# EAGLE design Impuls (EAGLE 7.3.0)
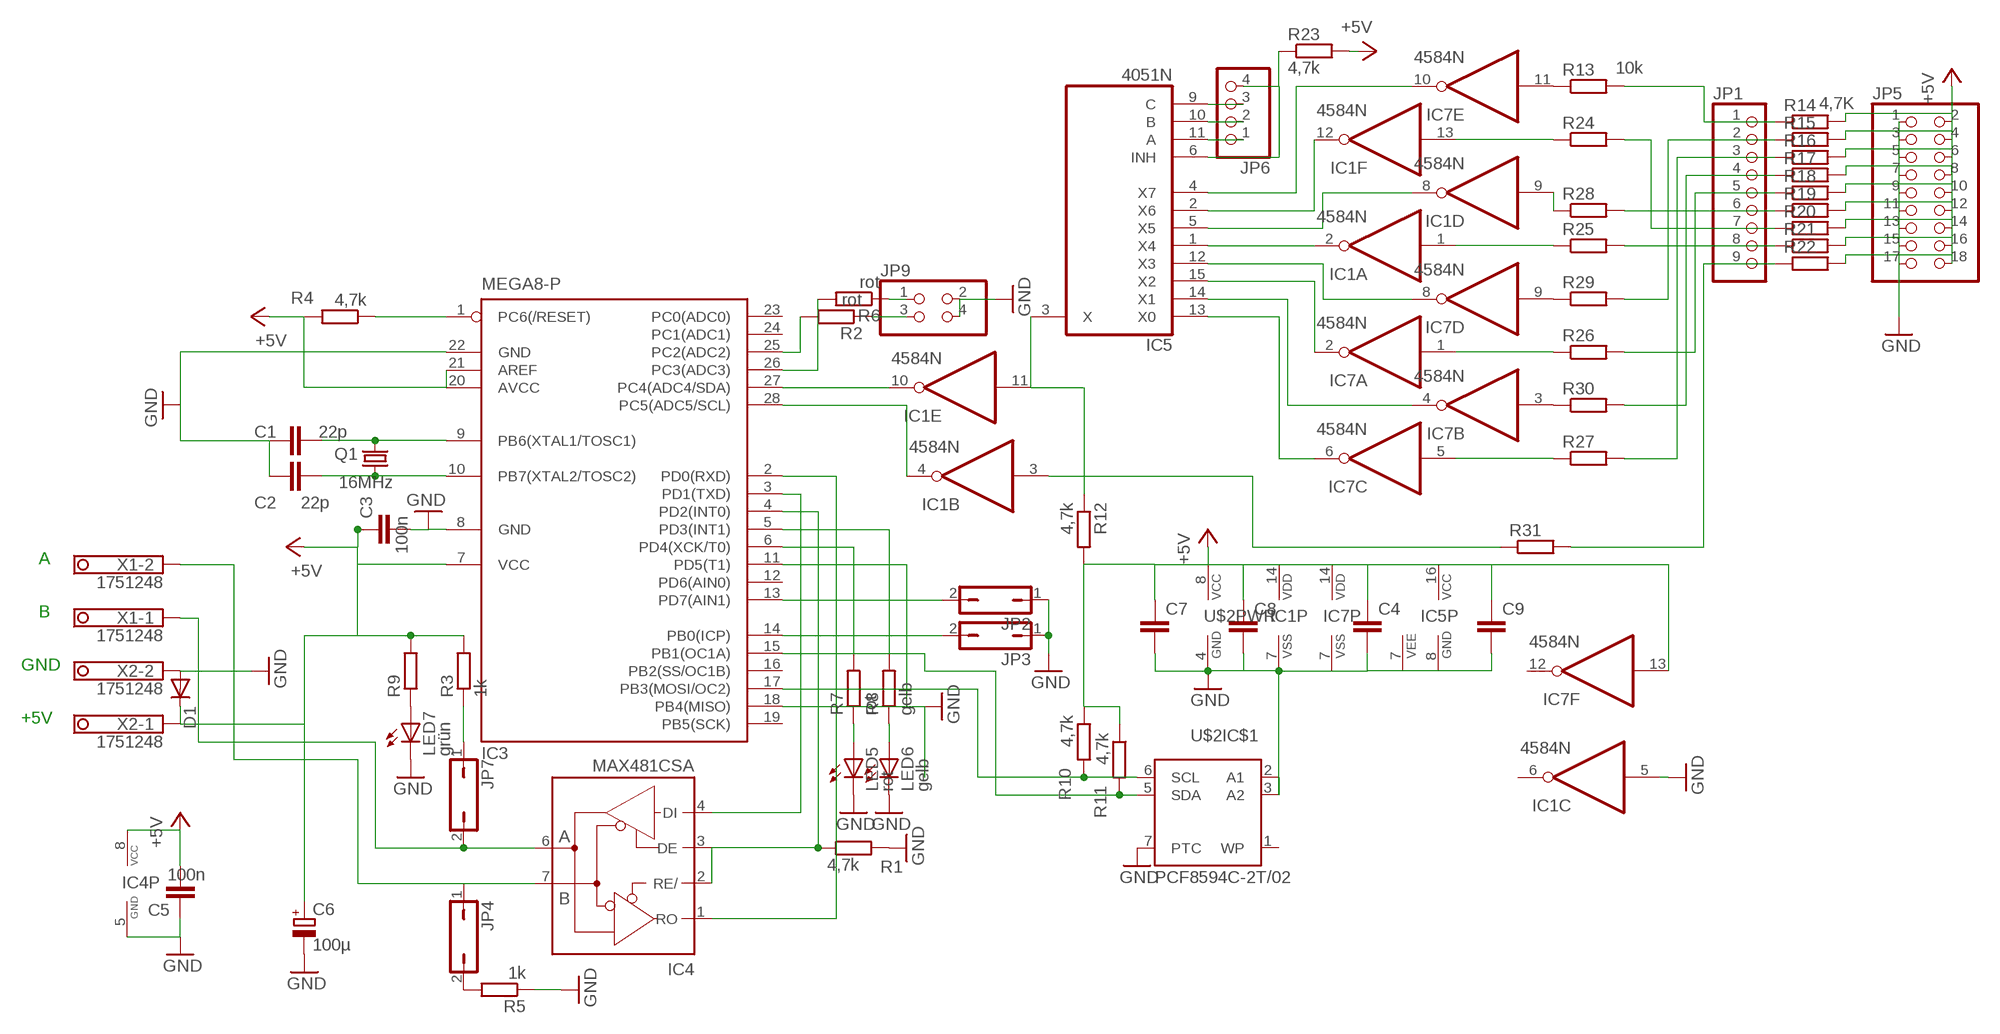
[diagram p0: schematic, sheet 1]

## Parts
C1  22p  C-EUC0603  [C0603]
C2  22p  C-EUC0603  [C0603]
C3  100n  C-EUC0603  [C0603]
C4  C-EUC0603  [C0603]
C5  100n  C-EUC0603  [C0603]
C6  100µ  CPOL-EUSMCD  [SMC_D]
C7  C-EUC0603  [C0603]
C8  C-EUC0603  [C0603]
C9  C-EUC0603  [C0603]
D1  DIODE-DO214AA  [DO214AA]
IC1  4584N  [DIL14]
IC3  MEGA8-P  [DIL28-3]
IC4  MAX481CSA  [SO08]
IC5  4051N  [DIL16]
IC7  4584N  [DIL14]
JP1  PINHD-1X9  [1X09]
JP2  JP1Q  [JP1]
JP3  JP1Q  [JP1]
JP4  JP1Q  [JP1]
JP5  PINHD-2X9  [2X09]
JP6  PINHD-1X4  [1X04]
JP7  JP1Q  [JP1]
JP9  PINHD-2X2  [2X02]
LED5  rot  LED3MM  [LED3MM]
LED6  gelb  LED3MM  [LED3MM]
LED7  grün  LED3MM  [LED3MM]
Q1  16MHz  CRYSTALCTS406  [CTS406]
R1  4,7k  R-EU_R0603  [R0603]
R2  rot  R-EU_R0603  [R0603]
R3  1k  R-EU_R0603  [R0603]
R4  4,7k  R-EU_R0603  [R0603]
R5  1k  R-EU_R0603  [R0603]
R6  rot  R-EU_R0603  [R0603]
R7  rot  R-EU_R0603  [R0603]
R8  gelb  R-EU_R0603  [R0603]
R9  R-EU_R0603  [R0603]
R10  4,7k  R-EU_R0603  [R0603]
R11  4,7k  R-EU_R0603  [R0603]
R12  4,7k  R-EU_R0603  [R0603]
R13  10k  R-EU_R0603  [R0603]
R14  4,7K  R-EU_R0603  [R0603]
R15  R-EU_R0603  [R0603]
R16  R-EU_R0603  [R0603]
R17  R-EU_R0603  [R0603]
R18  R-EU_R0603  [R0603]
R19  R-EU_R0603  [R0603]
R20  R-EU_R0603  [R0603]
R21  R-EU_R0603  [R0603]
R22  R-EU_R0603  [R0603]
R23  4,7k  R-EU_R0603  [R0603]
R24  R-EU_R0603  [R0603]
R25  R-EU_R0603  [R0603]
R26  R-EU_R0603  [R0603]
R27  R-EU_R0603  [R0603]
R28  R-EU_R0603  [R0603]
R29  R-EU_R0603  [R0603]
R30  R-EU_R0603  [R0603]
R31  R-EU_R0603  [R0603]
U$2  PCF8594C-2T/02  [SO08]
X1  1751248  [1751248]
X2  1751248  [1751248]

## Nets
+5V: C3.1 C4.1 C5.2 C6.+ C7.1 C8.1 C9.1 D1.C IC1.14(P:VDD) IC3.7(VCC) IC3.20(AVCC) IC3.21(AREF) IC4.8(VCC) IC5.16(VCC) IC7.13(F:I) IC7.14(P:VDD) JP5.2 JP5.4 JP5.6 JP5.8 JP5.10 JP5.12 JP5.14 JP5.16 JP5.18 R3.2 R4.2 R9.2 R10.1 R11.1 R12.2 R14.2 R15.2 R16.2 R17.2 R18.2 R19.2 R20.2 R21.2 R22.2 R23.2 U$2.8(PWR:VCC) X2.1
GND: C1.1 C2.1 C3.2 C4.2 C5.1 C6.- C7.2 C8.2 C9.2 D1.A IC1.5(C:I) IC1.7(P:VSS) IC3.8(GND) IC3.11(PD5(T1)) IC3.18(PB4(MISO)) IC3.22(GND) IC4.5(GND) IC5.7(VEE) IC5.8(GND) IC7.7(P:VSS) JP2.1 JP3.1 JP5.1 JP5.3 JP5.5 JP5.7 JP5.9 JP5.11 JP5.13 JP5.15 JP5.17 JP9.2 JP9.4 LED5.K(C) LED6.K(C) LED7.K(C) R1.2 R5.1 U$2.2(IC$1:A1) U$2.3(IC$1:A2) U$2.4(PWR:GND) U$2.7(IC$1:PTC) X2.2
N$1: IC1.4(B:O) IC3.28(PC5(ADC5/SCL))
N$2: IC3.2(PD0(RXD)) IC4.1(RO)
N$3: IC4.6(A) JP7.2 X1.1
N$4: IC4.7(B) JP4.1 X1.2
N$5: IC3.17(PB3(MOSI/OC2)) R10.2 U$2.6(IC$1:SCL)
N$6: IC3.13(PD7(AIN1)) JP2.2
N$7: IC3.15(PB1(OC1A)) R11.2 U$2.5(IC$1:SDA)
N$8: LED7.A R9.1
N$9: IC3.26(PC3(ADC3)) R6.2
N$10: IC3.1(PC6(/RESET)) R4.1
N$11: C2.2 IC3.10(PB7(XTAL2/TOSC2)) Q1.1
N$12: C1.2 IC3.9(PB6(XTAL1/TOSC1)) Q1.3
N$13: IC3.3(PD1(TXD)) IC4.4(DI)
N$14: IC3.14(PB0(ICP)) JP3.2
N$15: IC3.4(PD2(INT0)) IC4.2(RE/) IC4.3(DE) R1.1
N$16: IC3.25(PC2(ADC2)) R2.2
N$17: JP9.3 R2.1
N$18: JP9.1 R6.1
N$19: IC1.10(E:O) IC3.27(PC4(ADC4/SDA))
N$21: IC5.15(X2) IC7.2(A:O)
N$22: IC5.11(A) JP6.1
N$23: IC5.10(B) JP6.2
N$24: IC5.9(C) JP6.3
N$25: IC1.3(B:I) R31.1
N$26: IC1.2(A:O) IC5.1(X4)
N$27: IC1.12(F:O) IC5.2(X6)
N$28: IC1.8(D:O) IC5.5(X5)
N$29: IC5.4(X7) IC7.10(E:O)
N$30: IC5.13(X0) IC7.6(C:O)
N$31: IC5.14(X1) IC7.4(B:O)
N$32: JP1.8 R21.1 R25.2
N$33: IC5.12(X3) IC7.8(D:O)
N$34: IC1.11(E:I) IC5.3(X) R12.1
N$35: JP1.7 R20.1 R24.2
N$36: IC3.6(PD4(XCK/T0)) R7.2
N$37: IC3.5(PD3(INT1)) R8.2
N$38: LED5.A R7.1
N$39: LED6.A R8.1
N$40: JP1.6 R19.1 R28.2
N$41: JP1.5 R18.1 R26.2
N$42: JP1.4 R17.1 R30.2
N$43: IC1.9(D:I) R28.1
N$44: JP1.2 R15.1 R29.2
N$45: IC5.6(INH) JP6.4 R23.1
N$46: IC7.11(E:I) R13.1
N$47: IC1.13(F:I) R24.1
N$48: IC1.1(A:I) R25.1
N$49: IC7.1(A:I) R26.1
N$50: IC7.5(C:I) R27.1
N$51: JP1.3 R16.1 R27.2
N$52: IC7.3(B:I) R30.1
N$53: IC7.9(D:I) R29.1
N$54: JP1.9 R22.1 R31.2
N$55: JP1.1 R13.2 R14.1
N$56: JP4.2 R5.2
N$57: JP7.1 R3.1
Unconnected: IC1.6(C:O) IC3.12(PD6(AIN0)) IC3.16(PB2(SS/OC1B)) IC3.19(PB5(SCK)) IC3.23(PC0(ADC0)) IC3.24(PC1(ADC1)) IC7.12(F:O) U$2.1(IC$1:WP)

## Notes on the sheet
- A
- B
- GND
- +5V

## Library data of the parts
C1-C5 C7-C9 = rcl:C-EU: CAPACITOR, European symbol
C6 = rcl:CPOL-EU: POLARIZED CAPACITOR, European symbol
D1 = diode:DIODE-: DIODE
IC1 IC7 = 45xx:4584: Hex SCHMITT TRIGGER (74C14)
IC3 = atmel:MEGA8-P: MICROCONTROLLER 8 Kbytes FLASH, 1 kbytes SRAM, 512 bytes EEPROM, USART, 4-channel 10 bit ADC, 2-channel 8 bit ADC Pin compatible with Atmega48, ATMega88, ATMega168 Source: avr.lbr
IC4 = maxim:MAX481CSA: RS485 TRANSEIVER
IC5 = 40xx:4051: 8-channel ANALOG MULTIPLEXER
JP1 = pinhead:PINHD-1X9: PIN HEADER
JP2-JP4 JP7 = jumper:JP1Q: JUMPER
JP5 = pinhead:PINHD-2X9: PIN HEADER
JP6 = pinhead:PINHD-1X4: PIN HEADER
JP9 = pinhead:PINHD-2X2: PIN HEADER
LED5-LED7 = led:LED: LED
Q1 = crystal:CRYSTAL: CRYSTAL
R1-R31 = rcl:R-EU_: RESISTOR, European symbol
U$2 = i2c:PCF8594C-2: 512 x 8-Bit CMOS EEPROM with I²C Bus Interface
X1 X2 = con-phoenix-350:1751248: MKDS 1/ 2-3,5 Printklemme

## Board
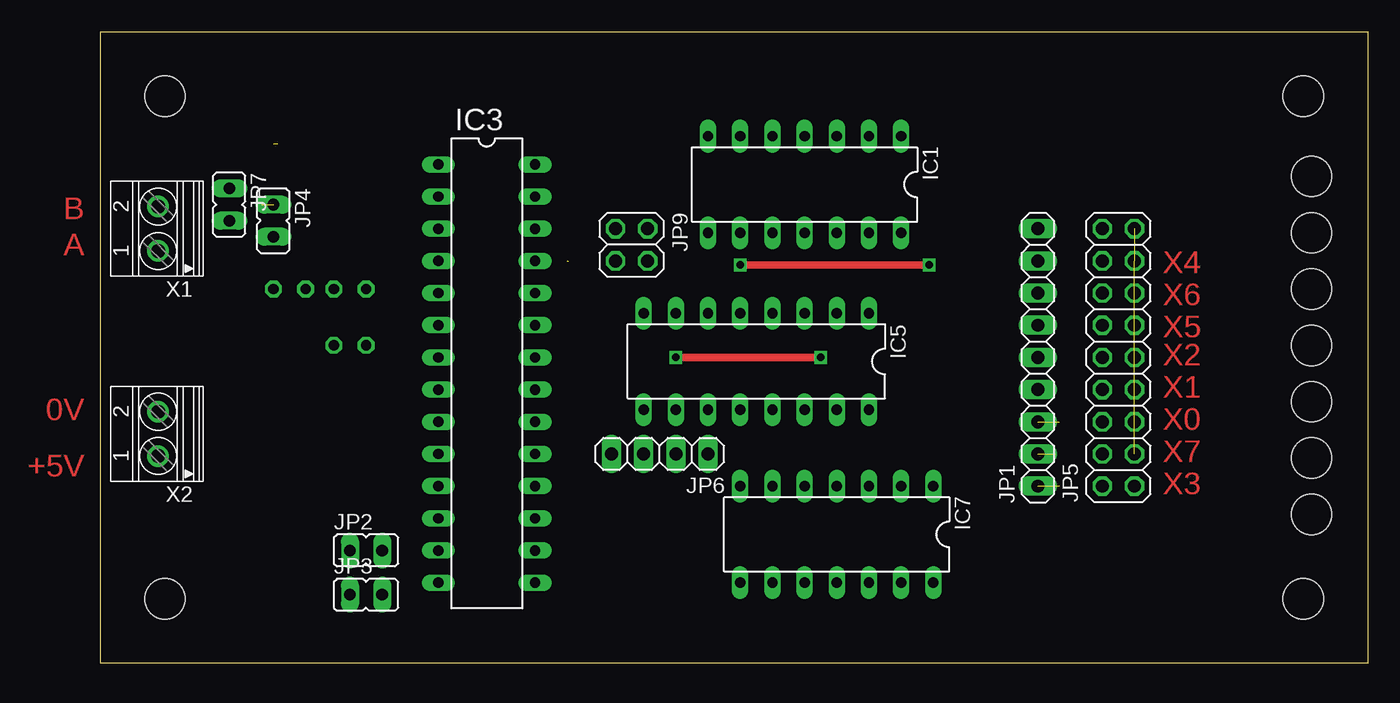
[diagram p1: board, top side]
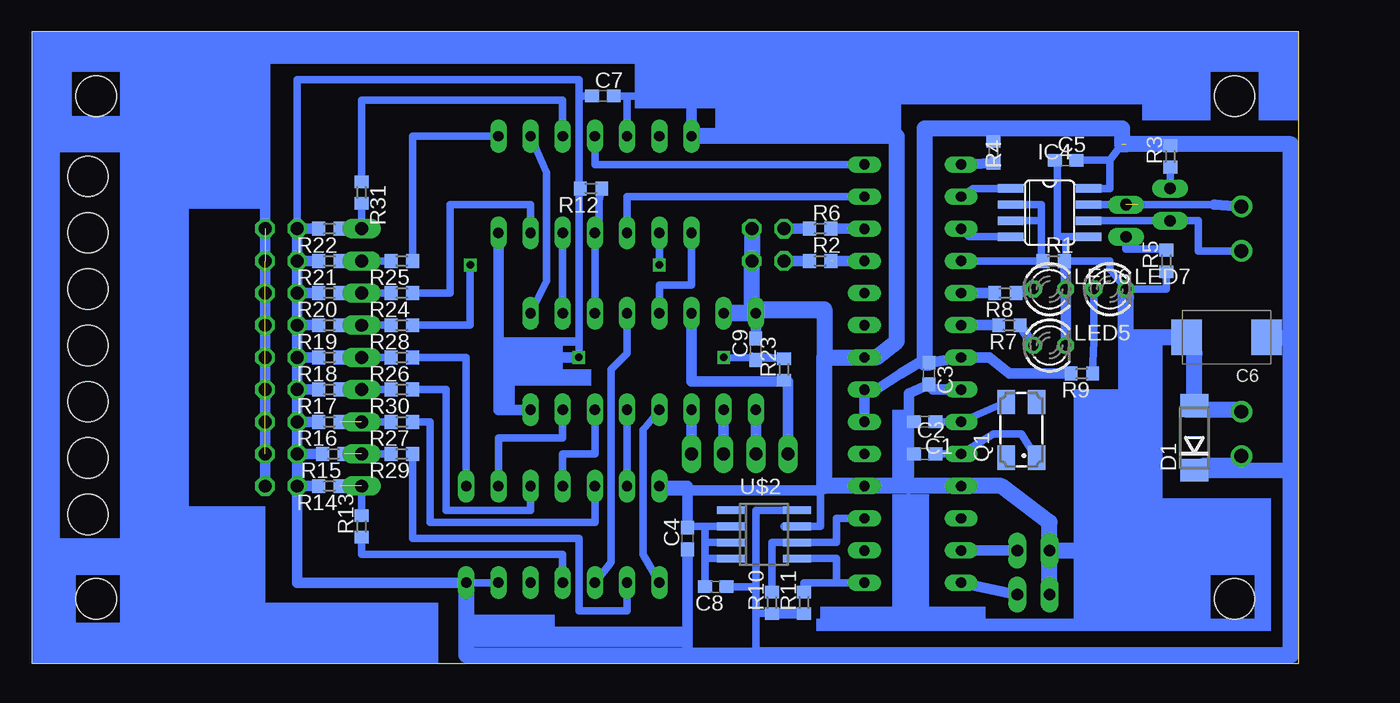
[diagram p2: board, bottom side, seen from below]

Size 100.01 x 49.85 mm. Coordinates in mm from the lower left corner, seen from the top.
Outline: 0,0 0,49.85 100.01,49.85 100.01,0 0,0
Copper layers (1*16): Top 0.035mm / dielectric 1.5mm / Bottom 0.035mm
Design rules "default": minimum track width 10mil, minimum drill 24mil, track to track 8mil, track to pad 8mil, pad to pad 8mil, via to via 8mil, smd to smd 8mil, copper to edge 40mil, drill to drill 8mil, minimum pad ring 10mil, minimum via ring 8mil, stop-mask expansion 4mil, vias tented up to drill 0mil, thermal gap 10mil
Holes 3.2 mm at 5.08,44.77 5.08,5.08 94.93,44.77 94.93,5.08 95.57,38.42 95.57,33.97 95.57,29.53 95.57,25.08 95.57,20.64 95.57,16.19 95.57,11.75

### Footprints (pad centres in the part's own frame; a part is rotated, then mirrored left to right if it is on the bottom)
C0603 = smd 1.1 x 1: 1 -0.85,0; 2 0.85,0
SMC_D = smd 2.4 x 2.8: + -3.15,0; - 3.15,0
DO214AA = smd 1.8 x 2.2: A 2.55,0; C -2.55,0
DIL14 = drill 0.813 long: 1 -7.62,-3.81; 2 -5.08,-3.81; 3 -2.54,-3.81; 4 0,-3.81; 5 2.54,-3.81; 6 5.08,-3.81; 7 7.62,-3.81; 8 7.62,3.81; 9 5.08,3.81; 10 2.54,3.81; 11 0,3.81; 12 -2.54,3.81; 13 -5.08,3.81; 14 -7.62,3.81
DIL28-3 = drill 0.813 long: 1 -16.51,-3.81; 2 -13.97,-3.81; 3 -11.43,-3.81; 4 -8.89,-3.81; 5 -6.35,-3.81; 6 -3.81,-3.81; 7 -1.27,-3.81; 8 1.27,-3.81; 9 3.81,-3.81; 10 6.35,-3.81; 11 8.89,-3.81; 12 11.43,-3.81; 13 13.97,-3.81; 14 16.51,-3.81; 15 16.51,3.81; 16 13.97,3.81; 17 11.43,3.81; 18 8.89,3.81; 19 6.35,3.81; 20 3.81,3.81; 21 1.27,3.81; 22 -1.27,3.81; 23 -3.81,3.81; 24 -6.35,3.81; 25 -8.89,3.81; 26 -11.43,3.81; 27 -13.97,3.81; 28 -16.51,3.81
SO08 = smd 0.66 x 2.032: 1 -1.905,-3.073; 2 -0.635,-3.073; 3 0.635,-3.073; 4 1.905,-3.073; 5 1.905,3.073; 6 0.635,3.073; 7 -0.635,3.073; 8 -1.905,3.073
DIL16 = drill 0.813 long: 1 -8.89,-3.81; 2 -6.35,-3.81; 3 -3.81,-3.81; 4 -1.27,-3.81; 5 1.27,-3.81; 6 3.81,-3.81; 7 6.35,-3.81; 8 8.89,-3.81; 9 8.89,3.81; 10 6.35,3.81; 11 3.81,3.81; 12 1.27,3.81; 13 -1.27,3.81; 14 -3.81,3.81; 15 -6.35,3.81; 16 -8.89,3.81
1X09 = drill 1.016 long: 1 -10.16,0; 2 -7.62,0; 3 -5.08,0; 4 -2.54,0; 5 0,0; 6 2.54,0; 7 5.08,0; 8 7.62,0; 9 10.16,0
JP1 = drill 0.914 long: 1 0,-1.27; 2 0,1.27
2X09 = drill 1.016 octagon: 1 -10.16,-1.27; 2 -10.16,1.27; 3 -7.62,-1.27; 4 -7.62,1.27; 5 -5.08,-1.27; 6 -5.08,1.27; 7 -2.54,-1.27; 8 -2.54,1.27; 9 0,-1.27; 10 0,1.27; 11 2.54,-1.27; 12 2.54,1.27; 13 5.08,-1.27; 14 5.08,1.27; 15 7.62,-1.27; 16 7.62,1.27; 17 10.16,-1.27; 18 10.16,1.27
1X04 = drill 1.016 long: 1 -3.81,0; 2 -1.27,0; 3 1.27,0; 4 3.81,0
2X02 = drill 1.016 octagon: 1 -1.27,-1.27; 2 -1.27,1.27; 3 1.27,-1.27; 4 1.27,1.27
LED3MM = drill 0.813 octagon: A -1.27,0; K 1.27,0
CTS406 = smd 1.9 x 1.4: 1 -2.2,-1.2; 2 2.2,-1.2; 3 2.2,1.2; 4 -2.2,1.2
R0603 = smd 1 x 1.1: 1 -0.85,0; 2 0.85,0
SO08' = smd 0.6 x 2.2: 1 -1.905,-2.6; 2 -0.635,-2.6; 3 0.635,-2.6; 4 1.905,-2.6; 5 1.905,2.6; 6 0.635,2.6; 7 -0.635,2.6; 8 -1.905,2.6
1751248 = drill 1.1 pad 1.7: 1 -1.75,-0.1; 2 1.75,-0.1

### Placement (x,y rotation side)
C1  29.53,19.05 0 bottom
C2  29.53,16.51 0 bottom
C3  29.21,22.86 270 bottom
C4  48.26,9.84 90 bottom
C5  18.41,39.69 0 bottom
C6  5.71,25.72 180 bottom
C7  54.93,44.77 0 bottom
C8  46.04,6.03 180 bottom
C9  42.86,24.77 90 bottom
D1  8.26,17.78 90 bottom
IC1  55.56,37.78 180 top
IC3  30.48,22.86 270 top
IC4  19.68,35.56 270 bottom
IC5  51.75,23.81 180 top
IC7  58.1,10.16 180 top
JP1  73.98,24.13 90 top
JP2  20.95,8.89 270 top
JP3  20.95,5.4 270 top
JP4  13.65,34.92 180 top
JP5  80.33,24.13 90 top
JP6  44.13,16.51 180 top
JP7  10.16,36.2 180 top
JP9  41.91,33.02 270 top
LED5  19.68,25.08 0 bottom
LED6  19.68,29.53 0 bottom
LED7  14.92,29.53 0 bottom
Q1  21.91,18.41 90 bottom
R1  19.37,31.75 0 bottom
R2  37.78,31.75 0 bottom
R3  10.16,40.01 90 bottom
R4  24.13,40.32 90 bottom
R5  10.48,31.75 90 bottom
R6  37.78,34.29 0 bottom
R7  22.86,26.67 180 bottom
R8  23.18,29.21 180 bottom
R9  17.14,22.86 180 bottom
R10  41.59,4.76 90 bottom
R11  39.05,4.76 90 bottom
R12  55.88,37.47 180 bottom
R13  73.98,10.79 90 bottom
R14  76.52,13.97 180 bottom
R15  76.2,16.51 180 bottom
R16  76.52,19.05 180 bottom
R17  76.52,21.59 180 bottom
R18  76.52,24.13 180 bottom
R19  76.52,26.67 180 bottom
R20  76.52,29.21 180 bottom
R21  76.52,31.75 180 bottom
R22  76.52,34.29 180 bottom
R23  40.64,23.18 90 bottom
R24  70.8,29.21 180 bottom
R25  70.8,31.75 180 bottom
R26  70.8,24.13 180 bottom
R27  70.8,19.05 180 bottom
R28  70.8,26.67 180 bottom
R29  70.8,16.51 180 bottom
R30  70.8,21.59 180 bottom
R31  73.98,37.15 270 bottom
U$2  PCF8594C-2T/02  [SO08']  42.23,10.16 270 bottom
X1  4.45,34.29 90 top
X2  4.45,18.1 90 top

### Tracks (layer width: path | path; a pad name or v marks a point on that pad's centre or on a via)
+5V  (via drill 0.6)  (1 unrouted)
  Top 0.61: v45.4,24.13 v56.83,24.13
  Bottom 0.61: IC4.8 14.92,37.47 14.92,39.69 | U$2.8 42.86,12.06 42.86,6.03 | 42.86,6.03 42.86,3.91 | 42.86,3.91 42.86,0.64 | C8.1 42.86,6.03 | R10.1 42.86,3.91 | R3.2 11.43,40.85 11.43,40.96 | C5.2 14.92,39.69 | 14.92,39.69 13.97,40.96 | v45.4,24.13 R23.2 43.18,24.23 C9.1 | R4.2 24.13,42.23 | v56.83,24.13 56.83,36.83 | 56.83,36.83 56.83,44.77 | 56.83,44.77 56.83,46.04 79.06,46.04 79.06,33.66 | C7.1 56.83,44.77 | R12.2 56.83,36.83 | IC7.13 IC7.14
  Bottom 0.813: IC3.20 IC3.21 33.34,21.59 31.43,22.86 29.84,23.81 C3.1 IC3.7 24.45,24.13 22.86,22.86 R9.2 | C4.1 48.26,0.64 | IC5.16 63.18,20 63.18,24.13 | 63.18,24.13 IC1.14 | v56.83,24.13 63.18,24.13 | JP5.16 79.06,33.66 JP5.18 R22.2 | JP5.16 JP5.14 | JP5.14 JP5.12 | JP5.12 JP5.10 | JP5.10 JP5.8 | JP5.8 JP5.6 | JP5.6 JP5.4 | JP5.4 JP5.2 | JP5.2 79.06,6.35 IC7.14 | R21.2 JP5.16 | R20.2 JP5.14 | R19.2 JP5.12 | R18.2 JP5.10 | R17.2 JP5.8 | R16.2 JP5.6 | R15.2 JP5.4 | JP5.2 R14.2 | R11.1 R10.1
  Bottom 1.27: 0.64,15.24 0.64,0.64 42.86,0.64 48.26,0.64 65.72,0.64 IC7.14 | 0.64,15.24 0.64,25.72 | 0.64,25.72 0.64,40.96 11.43,40.96 13.65,40.96 | 13.97,40.96 13.97,42.23 24.13,42.23 29.53,42.23 29.53,23.71 C3.1 | X2.1 5.08,15.56 7.62,15.56 D1.C 0.64,15.24 | C6.+ 0.64,25.72
GND  (7 unrouted)
  Bottom 0.61: IC4.5 18.41,33.66 | 18.41,33.66 18.41,32.38 R1.2 | C5.1 19.05,39.69 19.05,33.66 18.41,33.66 | R5.1 10.48,29.53 LED7.K 14.92,31.11 14.92,31.75 18.41,31.75 LED6.K | 40.64,10.79 U$2.7 37.78,10.79 37.78,13.65 37.47,14.29 | U$2.2 46.89,10.79 | 46.89,10.79 46.89,9.53 | 46.89,9.53 46.89,8.26 | 46.89,8.26 C8.2 | U$2.4 46.89,8.26 | U$2.3 46.89,9.53 | 46.89,10.79 48.26,10.79 C4.2 | C7.2 53.02,44.77 | 53.02,44.77 47.94,44.77 | C1.1 30.8,19.05 | C2.1 30.8,16.51 | IC1.5 53.02,44.77
  Bottom 0.813: LED5.K LED6.K 18.41,30.8 R1.2 | IC3.8 28.89,21.59 C3.2 30.8,21.27 30.8,19.05 30.8,16.51 30.8,13.97 | JP5.17 JP5.1 81.6,48.26 47.94,48.26 47.94,44.77 IC1.7 | C9.2 IC5.8 37.47,27.62 37.47,24.13 | C4.2 48.26,13.97 IC7.7 50.48,13.65 37.78,13.65
  Bottom 1.27: JP3.1 JP2.1 | JP2.1 13.65,8.89 13.65,25.72 | 13.65,28.89 LED7.K 13.65,25.72 | JP2.1 19.68,11.11 23.5,13.97 IC3.11 30.8,13.97 IC3.18 37.47,13.97 37.47,14.29 37.47,24.13 | X2.2 5.08,20 8.89,20 D1.A 8.26,24.45 C6.- 13.65,25.72 | IC5.8 IC5.7 43.18,27.62 43.18,27.94 | 43.18,27.94 JP9.4 JP9.2 | 43.18,27.94 37.47,27.94 37.47,24.13 | 37.47,24.13 IC3.22 33.34,24.13 31.75,25.4 31.75,41.59 IC1.7
N$1
  Bottom 0.61: IC3.28 55.56,39.37 IC1.4
N$2
  Bottom 0.61: IC4.1 25.72,37.47 IC3.2
N$3
  Bottom 0.61: IC4.6 15.88,34.92 11.43,34.92 JP7.2 7.94,34.92 7.94,32.54 X1.1
N$4  (1 unrouted)
  Bottom 0.61: 5.71,36.2 6.67,36.2 12.7,36.2 | JP4.1 IC4.7
  Bottom 0.813: X1.2 6.67,36.2
N$5
  Bottom 0.61: IC3.17 36.51,11.43 36.51,9.53 U$2.6 41.59,9.53 R10.2
N$6
  Bottom 0.813: JP2.2 IC3.13
N$7
  Bottom 0.61: U$2.5 36.51,8.26 36.51,6.35 | 36.51,6.35 IC3.15 | R11.2 39.05,6.35 36.51,6.35
N$8
  Bottom 0.61: LED7.A 16.19,25.4 R9.1
N$9
  Bottom 0.813: IC3.26 R6.2
N$10
  Bottom 0.813: R4.1 IC3.1
N$11
  Bottom 0.61: C2.2 IC3.10 24.13,18.1 21.91,18.1 Q1.1
N$12
  Bottom 0.61: Q1.3 IC3.9 C1.2
N$13
  Bottom 0.61: IC4.4 26.04,33.66 IC3.3
N$14
  Bottom 0.813: JP3.2 IC3.14
N$15
  Bottom 0.61: IC4.2 20.32,36.2 20.32,34.92 | IC3.4 R1.1 20.32,32.38 20.32,34.92 | IC4.3 20.32,34.92
N$16  (1 unrouted)
  Bottom 0.813: IC3.25 36.83,31.75
N$17
  Bottom 0.813: R2.1 JP9.3
N$18
  Bottom 0.813: R6.1 JP9.1
N$19
  Bottom 0.61: IC3.27 53.02,36.83 IC1.10
N$21
  Bottom 0.61: IC5.15 58.1,17.78 63.18,17.78 IC7.2
N$22
  Bottom 0.813: JP6.1 IC5.11
N$23
  Bottom 0.813: JP6.2 IC5.10
N$24
  Bottom 0.813: JP6.3 IC5.9
N$25
  Bottom 0.61: 58.2,41.59 IC1.3 58.1,44.45 73.98,44.45 R31.1
N$26
  Bottom 0.61: IC5.1 59.37,30.16 59.37,38.73 IC1.2
N$27
  Bottom 0.61: IC5.2 IC1.12
N$28
  Bottom 0.61: IC5.5 50.48,29.84 47.94,29.84 IC1.8
N$29
  Bottom 0.61: IC7.10 54.29,7.94 54.29,23.18 53.02,24.45 IC5.4
N$30
  Bottom 0.61: IC5.13 IC7.6
N$31
  Bottom 0.61: IC7.4 58.1,16.51 55.56,16.51 IC5.14
N$32
  Bottom 0.61: R21.1 JP1.8 R25.2
N$33
  Bottom 0.61: IC5.12 51.75,18.41 51.75,8.57 IC7.8
N$34
  Bottom 0.61: IC5.3 IC1.11 55.24,34.61 55.24,36.51 R12.1
N$35
  Bottom 0.61: R20.1 JP1.7 R24.2
N$36
  Bottom 0.813: R7.2 IC3.6
N$37
  Bottom 0.813: R8.2 IC3.5
N$38
  Bottom 0.813: LED5.A R7.1
N$39
  Bottom 0.813: LED6.A R8.1
N$40
  Bottom 0.61: R19.1 JP1.6 R28.2
N$41
  Bottom 0.61: R18.1 JP1.5 R26.2
N$42
  Bottom 0.61: R17.1 JP1.4 R30.2
N$43  (via drill 0.6)
  Top 0.61: v50.48,31.43 v65.41,31.43
  Bottom 0.61: IC1.9 v50.48,31.43 | v65.41,31.43 65.41,26.67 R28.1
N$44  (1 unrouted)
  Bottom 0.61: R29.2 JP1.2
N$45
  Bottom 0.61: R23.1 47.94,22.23
  Bottom 0.813: JP6.4 40.32,22.23 47.94,22.23 IC5.6
N$46
  Bottom 0.61: IC7.11 58.1,8.57 73.98,8.57 R13.1
N$47
  Bottom 0.61: IC1.13 60.64,36.2 66.99,36.2 66.99,29.21 R24.1
N$48
  Bottom 0.61: IC1.1 69.95,41.59 R25.1
N$49
  Bottom 0.61: IC7.1 65.72,24.13 R26.1
N$50
  Bottom 0.61: IC7.5 55.56,11.11 68.58,11.11 68.58,19.05 R27.1
N$51  (1 unrouted)
  Bottom 0.61: R27.2 JP1.3
N$52
  Bottom 0.61: IC7.3 60.64,12.06 67.31,12.06 67.31,21.59 R30.1
N$53
  Bottom 0.61: IC7.9 53.02,4.13 56.83,4.13 56.83,9.84 69.95,9.84 R29.1
N$54
  Bottom 0.61: R31.2 JP1.9 R22.1
N$55  (1 unrouted)
  Bottom 0.61: R13.2 JP1.1
N$56
  Bottom 0.61: JP4.2 13.65,32.7 10.48,32.7 R5.2
N$57
  Bottom 0.61: JP7.1 R3.1
(copper drawn outside any net)
  shapes: Bottom area x46

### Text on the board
Top: B | A | X4 | X6 | X5 | X2 | 0V | X1 | X0 | +5V | X7 | X3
